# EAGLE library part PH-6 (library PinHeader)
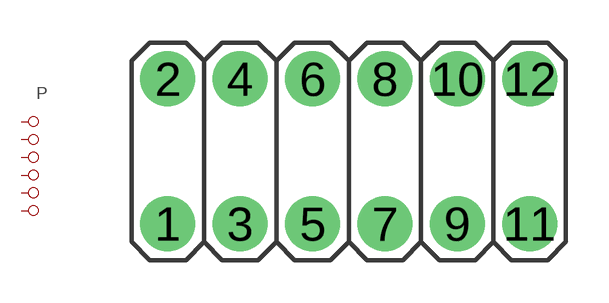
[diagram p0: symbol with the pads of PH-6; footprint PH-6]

Designator prefix P

## PH-6  [PH-6]
1  1  pas
2  1  pas
3  2  pas
4  2  pas
5  3  pas
6  3  pas
7  4  pas
8  4  pas
9  5  pas
10  5  pas
11  6  pas
12  6  pas

## Footprint PH-6 (pad centres in mm)
drill 1 pad 1.93: 1 -6.35,-2.54; 2 -6.35,2.54; 3 -3.81,-2.54; 4 -3.81,2.54; 5 -1.27,-2.54; 6 -1.27,2.54; 7 1.27,-2.54; 8 1.27,2.54; 9 3.81,-2.54; 10 3.81,2.54; 11 6.35,-2.54; 12 6.35,2.54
